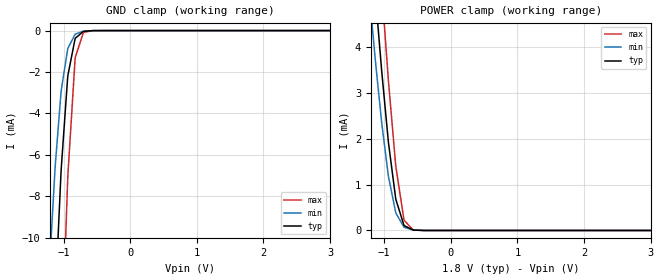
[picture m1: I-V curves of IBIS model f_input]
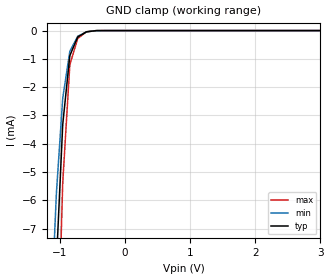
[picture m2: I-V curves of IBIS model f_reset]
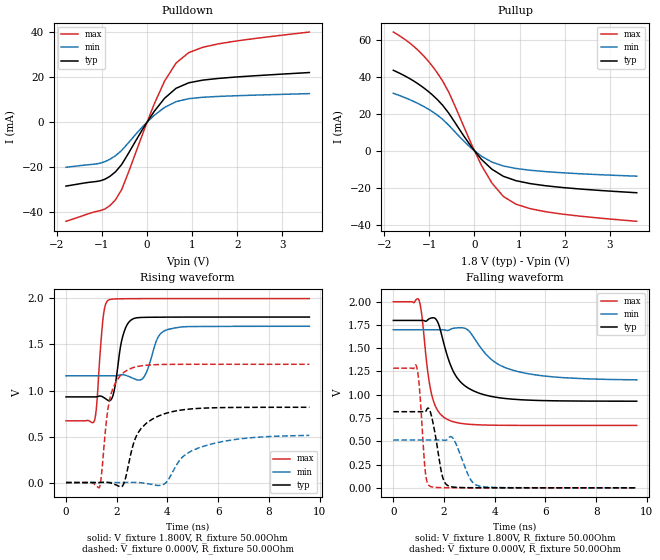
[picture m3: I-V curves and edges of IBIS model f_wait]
[IBIS Ver]   3.2
[File Name]   p30_18v_512m_65nm_b.ibs
[File Rev]   1.01
[Date]   9/9/2009
[Source]   From silicon level SPICE model at Numonyx B.V.
[Notes]   The following information corresponds to the 65nm P30
   512Mb chip with EzBGA package.
[Disclaimer]   This information is for modeling purposes only and is not
   guaranteed.Numonyx B.V. is not responsible for any problem
   this model may cause to customers.
[Copyright]   Copyright 2009, Numonyx B.V., All Rights Reserved.
[Component]   P30_18V_512M_EZBGA
[Manufacturer]  Numonyx B.V.
[Package]
|   typ   min   max
R_pkg   0.40Ohm   0.13Ohm   0.67Ohm
L_pkg   8.65nH   2.98nH   14.32nH
C_pkg   1.17pF   0.26pF   2.08pF
[PIN]   signal_name   model_name   R_pin   L_pin   C_pin
A1   A1   f_input   0.47   9.18nH   1.16pF
A2   A6   f_input   0.26   5.46nH   0.58pF
A3   A8   f_input   0.13   2.98nH   0.29pF
A4   VPP   POWER
A5   A13   f_input   0.28   5.89nH   0.66pF
A6   VCC   POWER
A7   A18   f_input   0.28   6.05nH   0.69pF
A8   A22   f_input   0.34   6.88nH   0.80pF
B1   A2   f_input   0.20   4.18nH   0.37pF
B2   VSS   GND
B3   A9   f_input   0.27   5.80nH   0.65pF
B4   CE#   f_input   0.45   8.83nH   1.10pF
B5   A14   f_input   0.28   5.89nH   0.65pF
B6   A25   f_input   0.52   9.67nH   1.22pF
B7   A19   f_input   0.45   8.60nH   1.16pF
B8   NC   NC
C1   A3   f_input   0.24   4.84nH   0.46pF
C2   A7   f_input   0.25   5.33nH   0.56pF
C3   A10   f_input   0.39   8.42nH   1.09pF
C4   A12   f_input   0.49   9.97nH   1.33pF
C5   A15   f_input   0.41   7.86nH   0.95pF
C6   WP#   f_input   0.26   5.46nH   0.59pF
C7   A20   f_input   0.47   8.74nH   1.15pF
C8   A21   f_input   0.28   5.82nH   0.63pF
D1   A4   f_input   0.29   6.08nH   0.68pF
D2   A5   f_input   0.25   5.17nH   0.53pF
D3   A11   f_input   0.55   9.98nH   1.26pF
D4   RST#   f_reset   0.35   6.81nH   0.77pF
D5   VCCQ   POWER
D6   VCCQ   POWER
D7   A16   f_input   0.30   5.86nH   0.70pF
D8   A17   f_input   0.33   6.41nH   0.70pF
E1   DQ8   f_inout   0.36   7.05nH   0.81pF
E2   DQ1   f_inout   0.33   6.32nH   0.69pF
E3   DQ9   f_inout   0.25   5.03nH   0.56pF
E4   DQ3   f_inout   0.25   5.00nH   0.55pF
E5   DQ4   f_inout   0.28   5.52nH   0.56pF
E6   CLK   f_input   0.27   5.42nH   0.55pF
E7   DQ15   f_inout   0.27   5.27nH   0.60pF
E8   NC   NC
F1   NC   NC
F2   DQ0   f_inout   0.24   4.94nH   0.57pF
F3   DQ10   f_inout   0.25   4.93nH   0.53pF
F4   DQ11   f_inout   0.20   4.19nH   0.43pF
F5   DQ12   f_inout   0.23   4.71nH   0.44pF
F6   ADV#   f_input   0.21   4.27nH   0.43pF
F7   WAIT   f_wait   0.23   4.62nH   0.51pF
F8   OE#   f_input   0.46   9.68nH   1.29pF
G1   A23   f_input   0.60   13.06nH   1.64pF
G2   NC   NC
G3   DQ2   f_inout   0.26   5.27nH   0.62pF
G4   VCCQ   POWER
G5   DQ5   f_inout   0.23   4.73nH   0.45pF
G6   DQ6   f_inout   0.25   5.05nH   0.49pF
G7   DQ14   f_inout   0.19   3.91nH   0.40pF
G8   WE#   f_input   0.46   9.41nH   1.10pF
H1   NC   NC
H2   VSS   GND
H3   VCC   POWER
H4   VSS   GND
H5   DQ13   f_inout   0.25   5.25nH   0.54pF
H6   VSSQ   GND
H7   DQ7   f_inout   0.13   2.99nH   0.26pF
H8   A24   f_input   0.67   14.32nH   2.08pF
| Models and submodels in the file (4): f_input (Input), f_reset (Input), f_wait (Output), f_inout (I/O)
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[Model]   f_input
Model_type   Input
Vinl = 0.400V
Vinh = 1.400V
|   typ   min   max
C_comp   4.280pF   2.270pF   4.770pF
[Voltage Range]   1.800V   1.700V   2.000V
[Temperature Range]   25.0   85.0   -40.0
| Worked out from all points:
|   GND clamp passes 1 mA (typ) near -0.86 V on its own axis
|   POWER clamp passes 1 mA (typ) near -0.85 V on its own axis
[GND Clamp]
|   Voltage   I(typ)   I(min)   I(max)
-1.8V     -80.25mA   -59.1mA    -114.4mA
-1.206V   -19.7mA    -11.07mA   -35.87mA
-1.152V   -15.16mA   -8.009mA   -29.37mA
-1.125V   -12.92mA   -6.504mA   -26.13mA
-1.093V   -10.64mA   -5.183mA   -22.51mA
-1.033V   -6.563mA   -2.845mA   -15.96mA
-941.4mV  -2.368mA   -948.8uA   -7.426mA
-828mV    -400.8uA   -185.4uA   -1.397mA
-822.6mV  -364.5uA   -170.8uA   -1.276mA
-703.8mV  -43.48uA   -28.19uA   -98.9uA
-563.4mV  -3.074uA   -3.137uA   -3.274uA
3.6V      0A         0A         0A
[POWER Clamp]
|   Voltage   I(typ)   I(min)   I(max)
-1.8V     18.62mA    15.61mA    22.69mA
-1.206V   6.51mA     4.864mA    8.909mA
-1.13V    5.103mA    3.675mA    7.246mA
-1.125V   5.004mA    3.592mA    7.129mA
-1.033V   3.407mA    2.296mA    5.183mA
-941.4mV  1.99mA     1.23mA     3.355mA
-828mV    699.7uA    395.3uA    1.428mA
-703.8mV  114.3uA    73.89uA    237.3uA
-698.4mV  105.3uA    68.73uA    218.4uA
-563.4mV  8.8uA      8.53uA     10.09uA
-412.2mV  495.2nA    779.4nA    260.9nA
3.6V      0A         0A         0A
[Model]   f_reset
Model_type   Input
Vinl = 0.400V
Vinh = 1.400V
|   typ   min   max
C_comp   2.570pF   1.290pF   2.610pF
[Voltage Range]   1.800V   1.700V   2.000V
[Temperature Range]   25.0   85.0   -40.0
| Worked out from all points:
|   GND clamp passes 1 mA (typ) near -0.85 V on its own axis
[GND Clamp]
|   Voltage   I(typ)   I(min)   I(max)
-1.8V     -77.85mA   -63.03mA   -101.5mA
-1.082V   -10.18mA   -7.202mA   -15.83mA
-1.076V   -9.791mA   -6.917mA   -15.29mA
-1.055V   -8.25mA    -5.779mA   -13.12mA
-1.033V   -7.154mA   -5.025mA   -11.41mA
-957.6mV  -3.346mA   -2.413mA   -5.432mA
-849.6mV  -921uA     -755.5uA   -1.269mA
-844.2mV  -866uA     -715.3uA   -1.181mA
-725.4mV  -224.5uA   -199.1uA   -275.8uA
-590.4mV  -43.29uA   -42.97uA   -41.36uA
-439.2mV  -1.59uA    -3.053uA   -485.9nA
3.6V      0A         0A         0A
[POWER Clamp]
|   Voltage   I(typ)   I(min)   I(max)
-1.8V     0A         0A         0A
0V        0A         0A         0A
1.699V    0A         0A         0A
1.802V    0A         0A         0A
2.002V    0A         0A         0A
3.6V      0A         0A         0A
[Model]   f_wait
Model_type   Output
Vmeas = 0.900V
Cref = 30.000pF
|   typ   min   max
C_comp   4.245pF   3.750pF   4.660pF
[Voltage Range]   1.800V   1.700V   2.000V
[Temperature Range]   25.0   85.0   -40.0
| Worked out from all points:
|   slope of the pulldown table from 0 to 0.27 V, typ, clamps not added: 35.4 ohm
|   slope of the pullup table from 0 to 0.27 V, typ, clamps not added: 36.9 ohm
|   falling waveform, V_fixture 1.800V, R_fixture 50.00Ohm: 20-80 % time 863ps typ, 1.44ns min, 405ps max; typ from 1.8 V to 0.931 V
|   rising waveform, V_fixture 1.800V, R_fixture 50.00Ohm: 20-80 % time 311ps typ, 390ps min, 206ps max; typ from 0.931 V to 1.8 V
|   rising waveform, V_fixture 0.000V, R_fixture 50.00Ohm: 20-80 % time 777ps typ, 1.44ns min, 402ps max; typ from 0.001 V to 0.818 V
|   falling waveform, V_fixture 0.000V, R_fixture 50.00Ohm: 20-80 % time 305ps typ, 451ps min, 189ps max; typ from 0.818 V to 0.001 V
[Pulldown]
|   Voltage   I(typ)   I(min)   I(max)
-1.8V     -28.37mA   -20.05mA   -43.95mA
-1.039V   -26.03mA   -18.22mA   -39.22mA
-828mV    -24.09mA   -16.53mA   -37.05mA
-703.8mV  -22.09mA   -14.96mA   -34.51mA
-563.4mV  -18.78mA   -12.55mA   -29.87mA
154.8mV   4.627mA    2.905mA    7.847mA
387mV     10.49mA    6.449mA    18.09mA
640.8mV   14.91mA    8.993mA    26.08mA
921.6mV   17.34mA    10.33mA    30.7mA
1.235V    18.54mA    10.95mA    33.08mA
1.575V    19.28mA    11.32mA    34.57mA
3.6V      21.9mA     12.57mA    39.83mA
[Pullup]
|   Voltage   I(typ)   I(min)   I(max)
-1.8V     43.58mA    31.16mA    64.26mA
-1.276V   36.67mA    25.93mA    54.98mA
-1.039V   32.45mA    22.83mA    48.95mA
-822.6mV  27.74mA    19.35mA    42.11mA
-563.4mV  20.18mA    13.73mA    31.41mA
-239.4mV  8.206mA    5.374mA    13.32mA
154.8mV   -4.549mA   -2.825mA   -7.796mA
387mV     -9.878mA   -6.007mA   -17.32mA
640.8mV   -13.7mA    -8.12mA    -24.59mA
921.6mV   -16.06mA   -9.455mA   -28.77mA
1.57V     -18.78mA   -11.15mA   -32.79mA
3.6V      -22.58mA   -13.63mA   -38mA
[Ramp]
R_load = 50.00Ohm
|   typ   min   max
dV/dt_r   490.132mV/776.470ps 307.117mV/1.439ns   770.276mV/402.058ps
dV/dt_f   519.915mV/862.419ps 322.660mV/1.433ns   795.985mV/405.316ps
[Falling Waveform]
V_fixture = 1.800V
V_fixture_min = 1.700V
V_fixture_max = 2.000V
R_fixture = 50.00Ohm
|   Time   V(typ)   V(min)   V(max)
0s        1.797V     1.698V     1.998V
1ns       1.797V     1.698V     2.023V
1.11ns    1.798V     1.698V     1.882V
1.51ns    1.824V     1.698V     1.004V
1.77ns    1.767V     1.698V     822.2mV
2.13ns    1.417V     1.689V     734.7mV
2.89ns    1.083V     1.704V     685.8mV
3.63ns    996.4mV    1.442V     675.1mV
5.25ns    943.5mV    1.229V     671.3mV
9.6ns     931mV      1.16V      671mV
[Rising Waveform]
V_fixture = 1.800V
V_fixture_min = 1.700V
V_fixture_max = 2.000V
R_fixture = 50.00Ohm
|   Time   V(typ)   V(min)   V(max)
0s        931mV      1.16V      671mV
1.12ns    930.9mV    1.16V      672.3mV
1.47ns    927.8mV    1.16V      1.804V
1.69ns    890.4mV    1.16V      1.984V
1.88ns    973.6mV    1.16V      1.993V
2.26ns    1.609V     1.171V     1.996V
2.65ns    1.778V     1.132V     1.997V
3.08ns    1.794V     1.149V     1.997V
4ns       1.797V     1.661V     1.998V
9.6ns     1.797V     1.698V     1.998V
[Rising Waveform]
V_fixture = 0.000V
V_fixture_min = 0.000V
V_fixture_max = 0.000V
R_fixture = 50.00Ohm
|   Time   V(typ)   V(min)   V(max)
0s        1.491mV    1.639mV    1.212mV
1.32ns    1.378mV    1.639mV    -49.42mV
1.61ns    3.706mV    1.642mV    707mV
1.75ns    -2.213mV   1.649mV    933.5mV
2.23ns    -34.79mV   2.092mV    1.183V
2.47ns    200.9mV    3.613mV    1.23V
2.97ns    591.5mV    -1.309mV   1.268V
3.88ns    747.7mV    -13.81mV   1.283V
5.25ns    806.5mV    379.2mV    1.285V
9.6ns     818.4mV    513.5mV    1.285V
[Falling Waveform]
V_fixture = 0.000V
V_fixture_min = 0.000V
V_fixture_max = 0.000V
R_fixture = 50.00Ohm
|   Time   V(typ)   V(min)   V(max)
0s        818.4mV    513.5mV    1.285V
910ps     818.4mV    513.5mV    1.308V
1.03ns    818.4mV    513.5mV    1.071V
1.26ns    816.5mV    513.5mV    176.4mV
1.46ns    815.2mV    513.5mV    16.46mV
1.92ns    142.1mV    513.7mV    3.011mV
2.2ns     19.27mV    542.7mV    2.093mV
3.03ns    2.868mV    97.3mV     1.371mV
3.36ns    2.319mV    22.61mV    1.295mV
9.6ns     1.491mV    1.639mV    1.212mV
